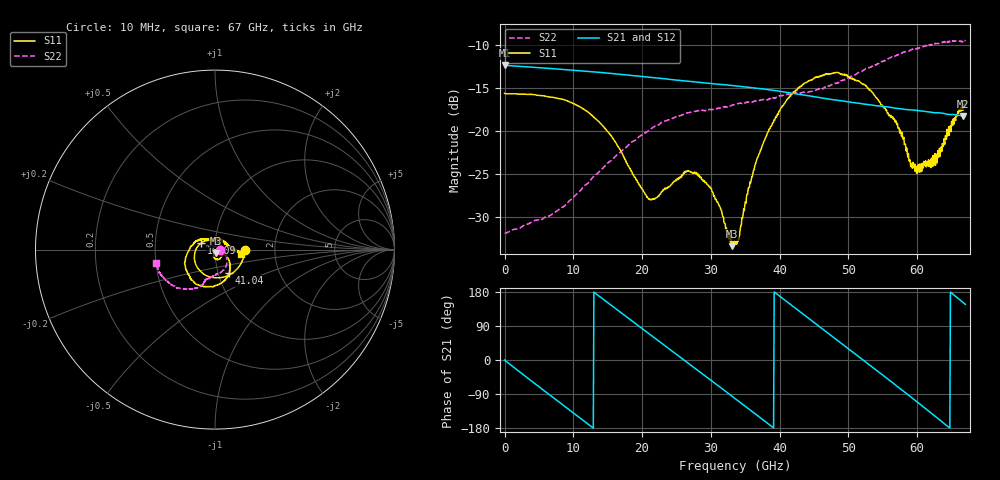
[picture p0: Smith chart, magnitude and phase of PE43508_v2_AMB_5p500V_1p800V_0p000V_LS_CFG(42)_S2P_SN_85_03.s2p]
!Keysight Technologies,N5227A,US51270237,A.10.43.00
!Date: Wednesday, August 22, 2018 17:10:57
!Correction: S11(Full 2 Port(1,3))
!S31(Full 2 Port(1,3))
!S13(Full 2 Port(1,3))
!S33(Full 2 Port(1,3))
!S2P File: Measurements: S11, S31, S13, S33:
# Hz S  dB  R 50
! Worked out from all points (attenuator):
!   801 points, 10 MHz to 67 GHz, reference 50 ohm
!   highest |S21| = -12.32 dB at 10 MHz (marker M1); lowest = -18.3 dB at 66.67 GHz (marker M2)
!   lowest |S11| = -33.4 dB at 33.09 GHz (marker M3), VSWR 1.04, Z = 50.4 - j2.1 ohm
!   |S11| at or under -10 dB: start of sweep to end of sweep
!   |S22| runs from -31.9 to -9.4 dB; largest |S21 - S12| = 0.0011
!   S11 on the Smith chart (normalised r, x): 10 MHz: 1.40, -0.00; 16.09 GHz: 0.85, +0.06; 41.04 GHz: 1.13, -0.30; 67 GHz: 1.34, -0.07
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1e7  -15.60 -0.4  -12.32 -0.2  -12.33 -0.2  -31.90 -0.6
5.787888e9  -15.92 -74.8  -12.66 -81.5  -12.66 -81.5  -30.12 -8.1
1.123082e10  -17.32 -140.9  -12.99 -156.7  -13.00 -156.7  -26.75 -16.6
1.60876e10  -21.30 155.6  -13.33 136.5  -13.33 136.5  -22.97 -30.1
2.07769e10  -27.73 57.8  -13.71 72.3  -13.71 72.3  -20.07 -48.1
2.236791e10  -27.61 10.4  -13.84 50.5  -13.84 50.6  -19.28 -55.1
2.638731e10  -24.79 -62.2  -14.17 -4.2  -14.17 -4.2  -17.91 -71.0
2.797832e10  -25.10 -77.5  -14.30 -25.9  -14.31 -25.9  -17.69 -76.0
3.01555e10  -27.05 -97.0  -14.48 -55.6  -14.48 -55.6  -17.52 -82.0
3.308631e10  -33.45 -78.6  -14.70 -95.8  -14.70 -95.7  -17.00 -89.3
3.3505e10  -33.19 -64.8  -14.73 -101.5  -14.74 -101.5  -16.93 -89.7
3.409116e10  -32.26 -46.7  -14.78 -109.6  -14.79 -109.6  -16.77 -90.6
3.668702e10  -23.29 -28.1  -15.02 -145.5  -15.02 -145.4  -16.46 -95.1
4.104138e10  -16.36 -58.4  -15.49 154.0  -15.50 154.1  -15.69 -101.4
4.472582e10  -14.01 -88.8  -15.94 103.0  -15.93 103.1  -15.38 -106.0
4.975008e10  -13.58 -130.2  -16.58 33.4  -16.57 33.4  -13.94 -109.1
5.251341e10  -14.75 -156.3  -16.88 -5.1  -16.87 -5.2  -12.74 -113.9
5.586291e10  -18.23 165.4  -17.20 -52.2  -17.20 -52.5  -11.52 -123.4
6.004979e10  -24.01 87.7  -17.62 -111.5  -17.63 -111.7  -10.40 -137.7
6.29806e10  -22.30 26.2  -17.87 -153.8  -17.89 -154.1  -9.81 -149.5
6.666505e10  -17.58 -7.8  -18.26 151.7  -18.32 151.8  -9.49 -165.0
6.7e10  -16.51 -9.6  -18.26 146.8  -18.32 146.8  -9.49 -167.2
